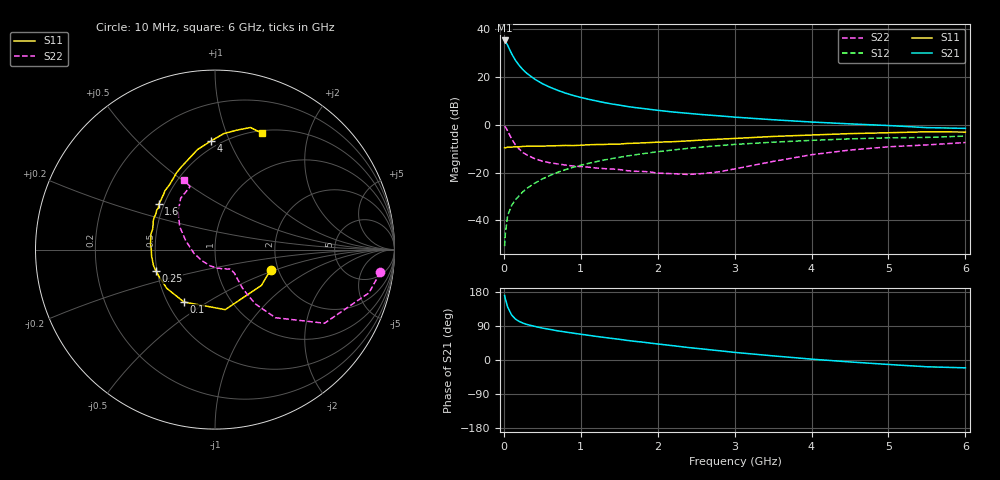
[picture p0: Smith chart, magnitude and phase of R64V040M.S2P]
! SIEMENS Small Signal Semiconductors
! BFR193
! Si NPN RF Bipolar Junction Transistor in SOT23
! VCE = 4 V  IC = 40 mA
! Common Emitter S-Parameters:  May  1996
# GHz  S  MA  R  50
!  f  S11  S21  S12  S22
! GHz  MAG  ANG  MAG  ANG  MAG  ANG  MAG  ANG
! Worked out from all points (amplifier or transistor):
!   36 points, 10 MHz to 6 GHz, reference 50 ohm
!   highest |S21| = 35.1 dB at 10 MHz (marker M1)
!   |S21| within 3 dB of that: start of sweep to 64.13 MHz
!   unconditionally stable (mu >= 1): 426.3 MHz to 1.917 GHz
!   at 250 MHz: K = 0.93, MSG = 25.4 dB, |S12| = -28.0 dB
!   at 1.4 GHz: K = 1.02, MAG = 10.6 dB, |S12| = -14.2 dB
!   at 6 GHz: K = 0.95, MSG = 1.6 dB, |S12| = -4.8 dB
!   S11 on the Smith chart (normalised r, x): 10 MHz: 1.83, -0.46; 100 MHz: 0.61, -0.40; 250 MHz: 0.49, -0.13; 1.6 GHz: 0.47, +0.29; 4 GHz: 0.45, +0.86; 6 GHz: 0.53, +1.34
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0.01  0.3297 -19.8  57.13 170.2  0.0029 86.2  0.9302 -7.8
0.02  0.3268 -37.6  55.04 161.0  0.0054 75.2  0.8909 -15.7
0.05  0.3393 -80.3  45.22 139.5  0.0127 70.8  0.7354 -33.9
0.1  0.3395 -120.6  30.48 119.1  0.0204 67.8  0.5076 -48.4
0.15  0.3446 -141.2  22.12 108.2  0.0269 68.6  0.3791 -53.3
0.2  0.3447 -152.0  17.18 101.7  0.0328 70.0  0.3078 -54.3
0.25  0.351 -160.6  13.91 97.2  0.04 71.7  0.2607 -54.4
0.3  0.354 -165.8  11.74 93.8  0.0467 72.4  0.2323 -53.6
0.4  0.3551 -174.4  8.927 88.8  0.0597 73.3  0.1951 -52.1
0.5  0.355 180.0  7.174 84.3  0.0733 73.5  0.1727 -50.7
0.6  0.3605 175.0  6.024 80.7  0.0869 72.9  0.1598 -50.7
0.7  0.363 170.1  5.197 77.0  0.1009 72.3  0.1512 -51.2
0.8  0.3676 166.1  4.557 73.9  0.1147 71.0  0.1432 -51.9
0.9  0.3653 162.0  4.071 70.9  0.1284 70.1  0.1365 -52.5
1.1  0.3794 155.1  3.388 65.2  0.155 67.7  0.1295 -57.3
1.6  0.4043 140.7  2.397 51.8  0.221 60.8  0.1094 -73.8
2.2  0.44 125.5  1.834 37.7  0.296 51.9  0.0945 -107.0
3.5  0.566 99.9  1.264 10.9  0.4301 31.6  0.1705 163.0
4  0.6064 92.0  1.133 2.3  0.4692 24.5  0.2354 146.8
4.5  0.6486 85.6  1.036 -5.1  0.5041 17.5  0.2946 134.1
5.5  0.7085 73.8  0.865 -17.9  0.5413 3.7  0.3769 111.6
6  0.6994 68.1  0.835 -20.7  0.5761 -0.3  0.4226 113.8
